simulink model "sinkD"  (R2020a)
settings: Solver=ode45  StartTime=0.0  StopTime=3000  RelTol=1e-3  EnableMultiTasking=on
InitFcn:
  | init_sink
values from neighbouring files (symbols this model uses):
  A = 0.1    [init_sink.m]    (also in init_waermeleit2.m = diag(-2*ones(N+1,1)) + diag(ones(N,1), 1) + diag(ones(N,1), )
  c1 = 1e7    (= 10000000)    [init_sink.m]    (also in init_waermeleit1.m = 0.002908; init_waermeleit2.m = 0.0727)
  c2 = 3e14    (= 300000000000000)    [init_sink.m]
  g = 9.81    [init_sink.m]
  rho = 1000    [init_sink.m]

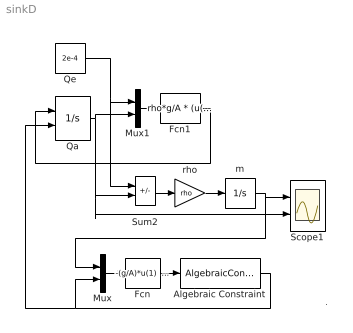
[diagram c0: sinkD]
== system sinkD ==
  note: .
  Algebraic Constraint : AlgebraicConstraint
  Fcn : Fcn  Expr="-(g/A)*u(1)  + c1*u(2) +c2*u(2)^3"
  Fcn1 : Fcn  Expr=rho*g/A * (u(1) - u(2)) / (c1 + 3*c2*u(2)^2)
  Mux : Mux  Inputs=2
  Mux1 : Mux  Inputs=2
  Qa : Integrator  InitialConditionSource=external  InitialCondition=0.0  LowerSaturationLimit=0
  Qe : Constant  Value=2e-4
  Scope1 : Scope  NumInputPorts=2
  Sum2 : Sum  Inputs=+-  SaturateOnIntegerOverflow=on
  m : Integrator  InitialCondition=10
  rho : Gain  Gain=rho
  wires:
  Qe/1 -> Mux1/1, Sum2/1
  Qa/1 -> Mux1/2, Sum2/2, Scope1/2
  Mux1/1 -> Fcn1/1
  Fcn1/1 -> Qa/1
  Sum2/1 -> rho/1
  m/1 -> Mux/1, Scope1/1
  Mux/1 -> Fcn/1
  Fcn/1 -> Algebraic Constraint/1
  Algebraic Constraint/1 -> Qa/2, Mux/2
  rho/1 -> m/1
